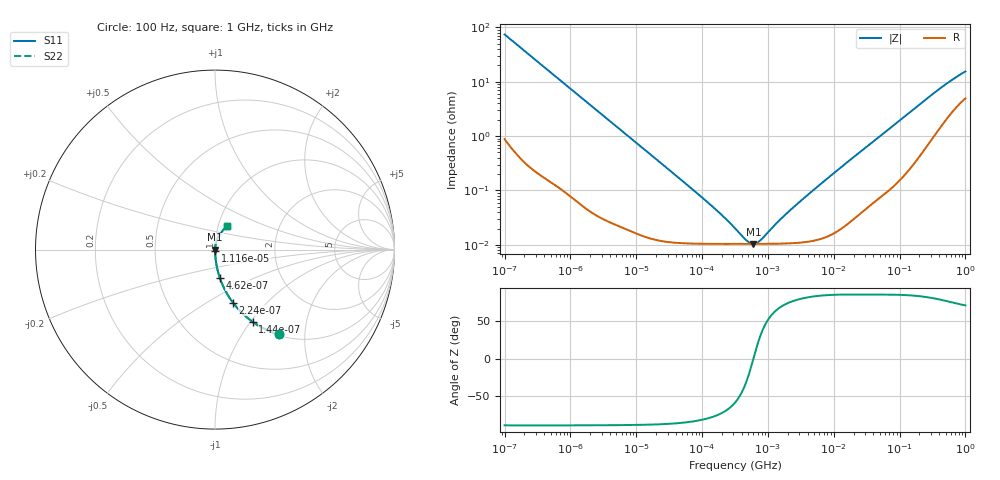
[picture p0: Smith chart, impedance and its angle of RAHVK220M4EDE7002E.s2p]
! RAHVK220M4EDE7002E  S-PARAMETER MODEL  (AEC-Q200 qualified)
! Model Generated by ELNA Corporation (http://www.ty-top.com)
! Version 1.0
! ELNA Control No. 201214
! Copyright (c) 2020 ELNA CO.,LTD. All Rights Reserved.
! Products Name : CONDUCTIVE POLYMER HYBRID ALUMINUM ELECTROLYTIC CAPACITORS
! Characteristics :
!  Capacitance  :  22uF  ,  Rated voltage  :  63V
!  Operating Temp. Range  :  -55 to +125 degC  ,  Endurance  :  4000hr at 125 degC
!  Dimension D  :  6.3mm  ,  Dimension L  :  7.7mm
! Frequency Range : 100Hz - 1GHz
! External Node Assignments :
!  1  o---| |---o  2
# MHz S RI R 50
!Freq[MHz].  S11 Real  S11 Imag  S21 Real  S21 Imag  S12 Real  S12 Imag  S22 Real  S22 Imag
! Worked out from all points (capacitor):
!   401 points, 100 Hz to 1 GHz, reference 50 ohm
!   read as one part in series: C = 21.6 uF near 108 Hz
!   lowest |Z| = 10.4 mohm at 602.6 kHz (marker M1)
!   series resonance near 601.6 kHz, so ESL is about 3.2 nH
!   S11 on the Smith chart (normalised r, x): 100 Hz: 1.02, -1.47; 144 Hz: 1.01, -1.03; 224 Hz: 1.01, -0.66; 462 Hz: 1.00, -0.32; 11.16 kHz: 1.00, -0.01; 1 GHz: 1.10, +0.29
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0.0001  0.3539 -0.4723  0.6461 0.4723  0.6461 0.4723  0.3539 -0.4723
0.000144  0.2108 -0.403  0.7892 0.403  0.7892 0.403  0.2108 -0.403
0.000224  0.1001 -0.2958  0.8999 0.2958  0.8999 0.2958  0.1001 -0.2958
0.000462  0.0264 -0.1556  0.9736 0.1556  0.9736 0.1556  0.0264 -0.1556
0.000781  0.00991 -0.0941  0.9901 0.0941  0.9901 0.0941  0.00991 -0.0941
0.001488  0.00303 -0.0499  0.997 0.0499  0.997 0.0499  0.00303 -0.0499
0.011156  0.000199 -0.00675  0.9998 0.00675  0.9998 0.00675  0.000199 -0.00675
0.022131  0.000132 -0.00341  0.9999 0.00341  0.9999 0.00341  0.000132 -0.00341
0.130317  0.000105 -0.000554  0.9999 0.000554  0.9999 0.000554  0.000105 -0.000554
0.211349  0.000104 -0.000314  0.9999 0.000314  0.9999 0.000314  0.000104 -0.000314
0.316228  0.000104 -0.000173  0.9999 0.000173  0.9999 0.000173  0.000104 -0.000173
0.473151  0.000104 -6.1e-05  0.9999 6.1e-05  0.9999 6.1e-05  0.000104 -6.1e-05
0.533949  0.000104 -3.01e-05  0.9999 3.01e-05  0.9999 3.01e-05  0.000104 -3.01e-05
0.60256  0.000104 4.02e-07  0.9999 -4.02e-07  0.9999 -4.02e-07  0.000104 4.02e-07
0.679986  0.000104 3.09e-05  0.9999 -3.09e-05  0.9999 -3.09e-05  0.000104 3.09e-05
0.767361  0.000104 6.19e-05  0.9999 -6.19e-05  0.9999 -6.19e-05  0.000104 6.19e-05
1.788546  0.000106 0.000332  0.9999 -0.000332  0.9999 -0.000332  0.000106 0.000332
4.704354  0.000119 0.000966  0.9999 -0.000966  0.9999 -0.000966  0.000119 0.000966
69.9842  0.0012 0.0136  0.9988 -0.0136  0.9988 -0.0136  0.0012 0.0136
395.8221  0.0179 0.0691  0.9821 -0.0691  0.9821 -0.0691  0.0179 0.0691
668.3439  0.04 0.1024  0.96 -0.1024  0.96 -0.1024  0.04 0.1024
1000  0.0652 0.1302  0.9348 -0.1302  0.9348 -0.1302  0.0652 0.1302
